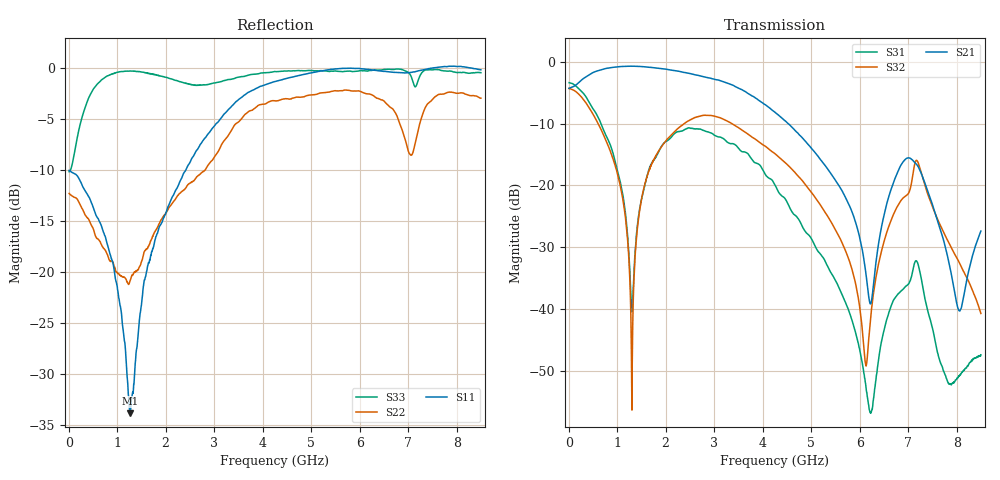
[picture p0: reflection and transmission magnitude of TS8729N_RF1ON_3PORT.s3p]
!Created with skrf (http://scikit-rf.org).
# GHz S RI R 50.0
!freq ReS11 ImS11 ReS12 ImS12 ReS13 ImS13
! ReS21 ImS21 ReS22 ImS22 ReS23 ImS23
! ReS31 ImS31 ReS32 ImS32 ReS33 ImS33
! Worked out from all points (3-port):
!   1601 points, 10 MHz to 8.5 GHz, reference 50 ohm
!   strongest paths, dB at 10 MHz, 2.132 GHz, 4.255 GHz, 6.378 GHz, 8.5 GHz:
!     S21: -4.3, -1.4, -8.2, -30.1, -27.4
!     S32: -4.3, -11.7, -14.9, -33.2, -40.7
!     S31: -3.4, -12.0, -19.9, -48.8, -47.4
!   lowest |S11| = -33.9 dB at 1.262 GHz (marker M1), VSWR 1.04, Z = 49.6 + j1.98 ohm
!   |S11| at or under -10 dB: start of sweep to 2.414 GHz
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0.01  -0.3157 0.0163  0.6114 0.00626  0.6778 -0.0183
      0.6114 0.00605  -0.2429 0.0129  0.6072 -0.0161
      0.6777 -0.0186  0.6074 -0.016  -0.3092 0.0364
0.6785875  0.0299 0.1652  0.8416 -0.2044  -0.00284 -0.3079
           0.8412 -0.2044  0.0303 0.1328  0.0321 -0.2761
           -0.00265 -0.308  0.032 -0.2763  0.8726 0.1026
1.262275  -0.00367 0.0199  0.6972 -0.603  -0.00908 -0.0178
          0.6971 -0.6028  0.086 -0.0267  -0.00988 -0.0141
          -0.00913 -0.0179  -0.00977 -0.0141  0.5164 -0.8229
2.365975  -0.0579 0.2984  -0.00204 -0.8235  0.107 -0.2585
          -0.00265 -0.8227  -0.0579 -0.2458  0.2472 -0.1913
          0.1069 -0.258  0.2476 -0.191  -0.8518 -0.0187
4.255  0.7689 0.3899  -0.3912 -0.0103  -0.0857 0.0531
       -0.3902 -0.00985  -0.6298 0.2913  -0.1773 -0.0308
       -0.0857 0.0528  -0.1778 -0.0312  0.7734 0.5775
6.218312  0.9762 -0.1439  -0.0108 -0.00225  -0.00142 0.000262
          -0.0108 -0.00229  0.4598 0.5885  -0.00101 -0.00781
          -0.00142 0.000271  -0.00103 -0.00783  0.9733 -0.0909
6.897513  0.9012 -0.3071  -0.1244 -0.0939  -0.0125 -0.00725
          -0.1243 -0.0933  0.1642 -0.4532  -0.0502 -0.061
          -0.0126 -0.00717  -0.0501 -0.0613  0.9283 -0.3246
7.178744  0.9244 -0.2857  -0.1448 0.0265  -0.0239 0.00439
          -0.1452 0.0266  -0.4151 0.2033  -0.1572 -0.0267
          -0.0239 0.00434  -0.1569 -0.0267  0.8114 -0.1945
8.048969  1.002 -0.198  -0.00962 -0.0017  -0.00264 -0.00112
          -0.00955 -0.00167  0.4697 0.5924  -0.011 0.0212
          -0.00262 -0.00118  -0.011 0.0213  0.9278 -0.225
8.5  0.9268 -0.3321  -0.0104 -0.0414  -0.00347 -0.00242
     -0.0105 -0.0414  0.6124 0.3683  -0.00478 0.00784
     -0.00348 -0.00245  -0.00483 0.00782  0.907 -0.2921
